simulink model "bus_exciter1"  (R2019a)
settings: Solver=VariableStepAuto  StartTime=0.0  StopTime=10.0  RelTol=1e-3
undefined symbols (not defined in the file or in its folder): DiscIntNeverNeededParam, sig1, sig2, subbus1, subbus2

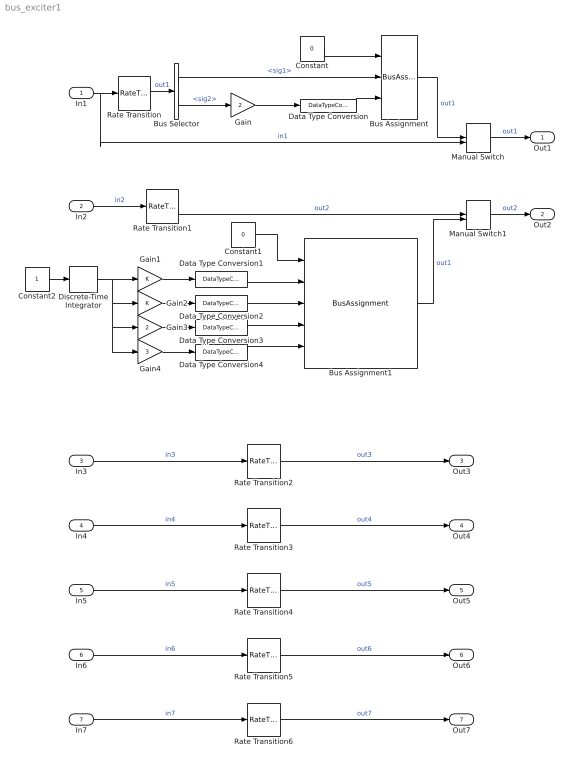
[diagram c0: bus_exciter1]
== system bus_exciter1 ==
  In1 : Inport  OutDataTypeStr=Bus: bus1
  In2 : Inport  Port=2  OutDataTypeStr=Bus: bus3
  In3 : Inport  Port=3  OutDataTypeStr=single  PortDimensions=1
  In4 : Inport  Port=4  OutDataTypeStr=single  PortDimensions=4
  In5 : Inport  Port=5  OutDataTypeStr=Bus: bus4  PortDimensions=1
  In6 : Inport  Port=6  OutDataTypeStr=Bus: bus2  PortDimensions=2
  In7 : Inport  Port=7  OutDataTypeStr=Bus: bus2  PortDimensions=2
  Bus Assignment : BusAssignment  AssignedSignals=sig1,sig2
  Bus Assignment1 : BusAssignment  AssignedSignals=subbus1.sig1,subbus1.sig2,subbus2.sig1,subbus2.sig2
  Bus Selector : BusSelector  OutputSignals=sig1,sig2
  Constant : Constant  Value=0  OutDataTypeStr=Bus: bus1
  Constant1 : Constant  Value=0  OutDataTypeStr=Bus: bus3
  Constant2 : Constant  OutDataTypeStr=single
  Data Type Conversion : DataTypeConversion  OutDataTypeStr=uint8
  Data Type Conversion{1..4} (4 alike) : DataTypeConversion
  Discrete-Time Integrator : DiscreteIntegrator  SampleTime=-1  ICPrevOutput=DiscIntNeverNeededParam  ICPrevScaledInput=DiscIntNeverNeededParam
  Gain : Gain  Gain=2
  Gain1 : Gain
  Gain2 : Gain
  Gain3 : Gain  Gain=2
  Gain4 : Gain  Gain=3
  Manual Switch : ManualSwitch  CurrentSetting=0
  Manual Switch1 : ManualSwitch  CurrentSetting=0
  Rate Transition{,1..6} (7 alike) : RateTransition
  Out1 : Outport  OutDataTypeStr=Bus: bus1
  Out2 : Outport  Port=2  OutDataTypeStr=Bus: bus3
  Out3 : Outport  Port=3  OutDataTypeStr=single  PortDimensions=1
  Out4 : Outport  Port=4  OutDataTypeStr=single  PortDimensions=4
  Out5 : Outport  Port=5  OutDataTypeStr=Bus: bus4
  Out6 : Outport  Port=6  OutDataTypeStr=Bus: bus2  PortDimensions=2
  Out7 : Outport  Port=7  OutDataTypeStr=Bus: bus2  PortDimensions=2
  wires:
  In1/1 -> Manual Switch/2, Rate Transition/1  "in1"
  In2/1 -> Rate Transition1/1  "in2"
  In3/1 -> Rate Transition2/1  "in3"
  In4/1 -> Rate Transition3/1  "in4"
  In5/1 -> Rate Transition4/1  "in5"
  In6/1 -> Rate Transition5/1  "in6"
  Manual Switch/1 -> Out1/1  "out1"
  Manual Switch1/1 -> Out2/1  "out2"
  Rate Transition2/1 -> Out3/1  "out3"
  Rate Transition3/1 -> Out4/1  "out4"
  Rate Transition4/1 -> Out5/1  "out5"
  Rate Transition5/1 -> Out6/1  "out6"
  Constant/1 -> Bus Assignment/1
  Rate Transition/1 -> Bus Selector/1  "out1"
  Bus Selector/1 -> Bus Assignment/2  "<sig1>"
  Bus Selector/2 -> Gain/1  "<sig2>"
  Gain/1 -> Data Type Conversion/1
  Data Type Conversion/1 -> Bus Assignment/3
  Bus Assignment/1 -> Manual Switch/1  "out1"
  In7/1 -> Rate Transition6/1  "in7"
  Rate Transition6/1 -> Out7/1  "out7"
  Rate Transition1/1 -> Manual Switch1/1  "out2"
  Constant1/1 -> Bus Assignment1/1
  Bus Assignment1/1 -> Manual Switch1/2  "out1"
  Constant2/1 -> Discrete-Time Integrator/1
  Discrete-Time Integrator/1 -> Gain4/1, Gain3/1, Gain2/1, Gain1/1
  Gain1/1 -> Data Type Conversion1/1
  Gain2/1 -> Data Type Conversion2/1
  Gain3/1 -> Data Type Conversion3/1
  Gain4/1 -> Data Type Conversion4/1
  Data Type Conversion1/1 -> Bus Assignment1/2
  Data Type Conversion2/1 -> Bus Assignment1/3
  Data Type Conversion3/1 -> Bus Assignment1/4
  Data Type Conversion4/1 -> Bus Assignment1/5
